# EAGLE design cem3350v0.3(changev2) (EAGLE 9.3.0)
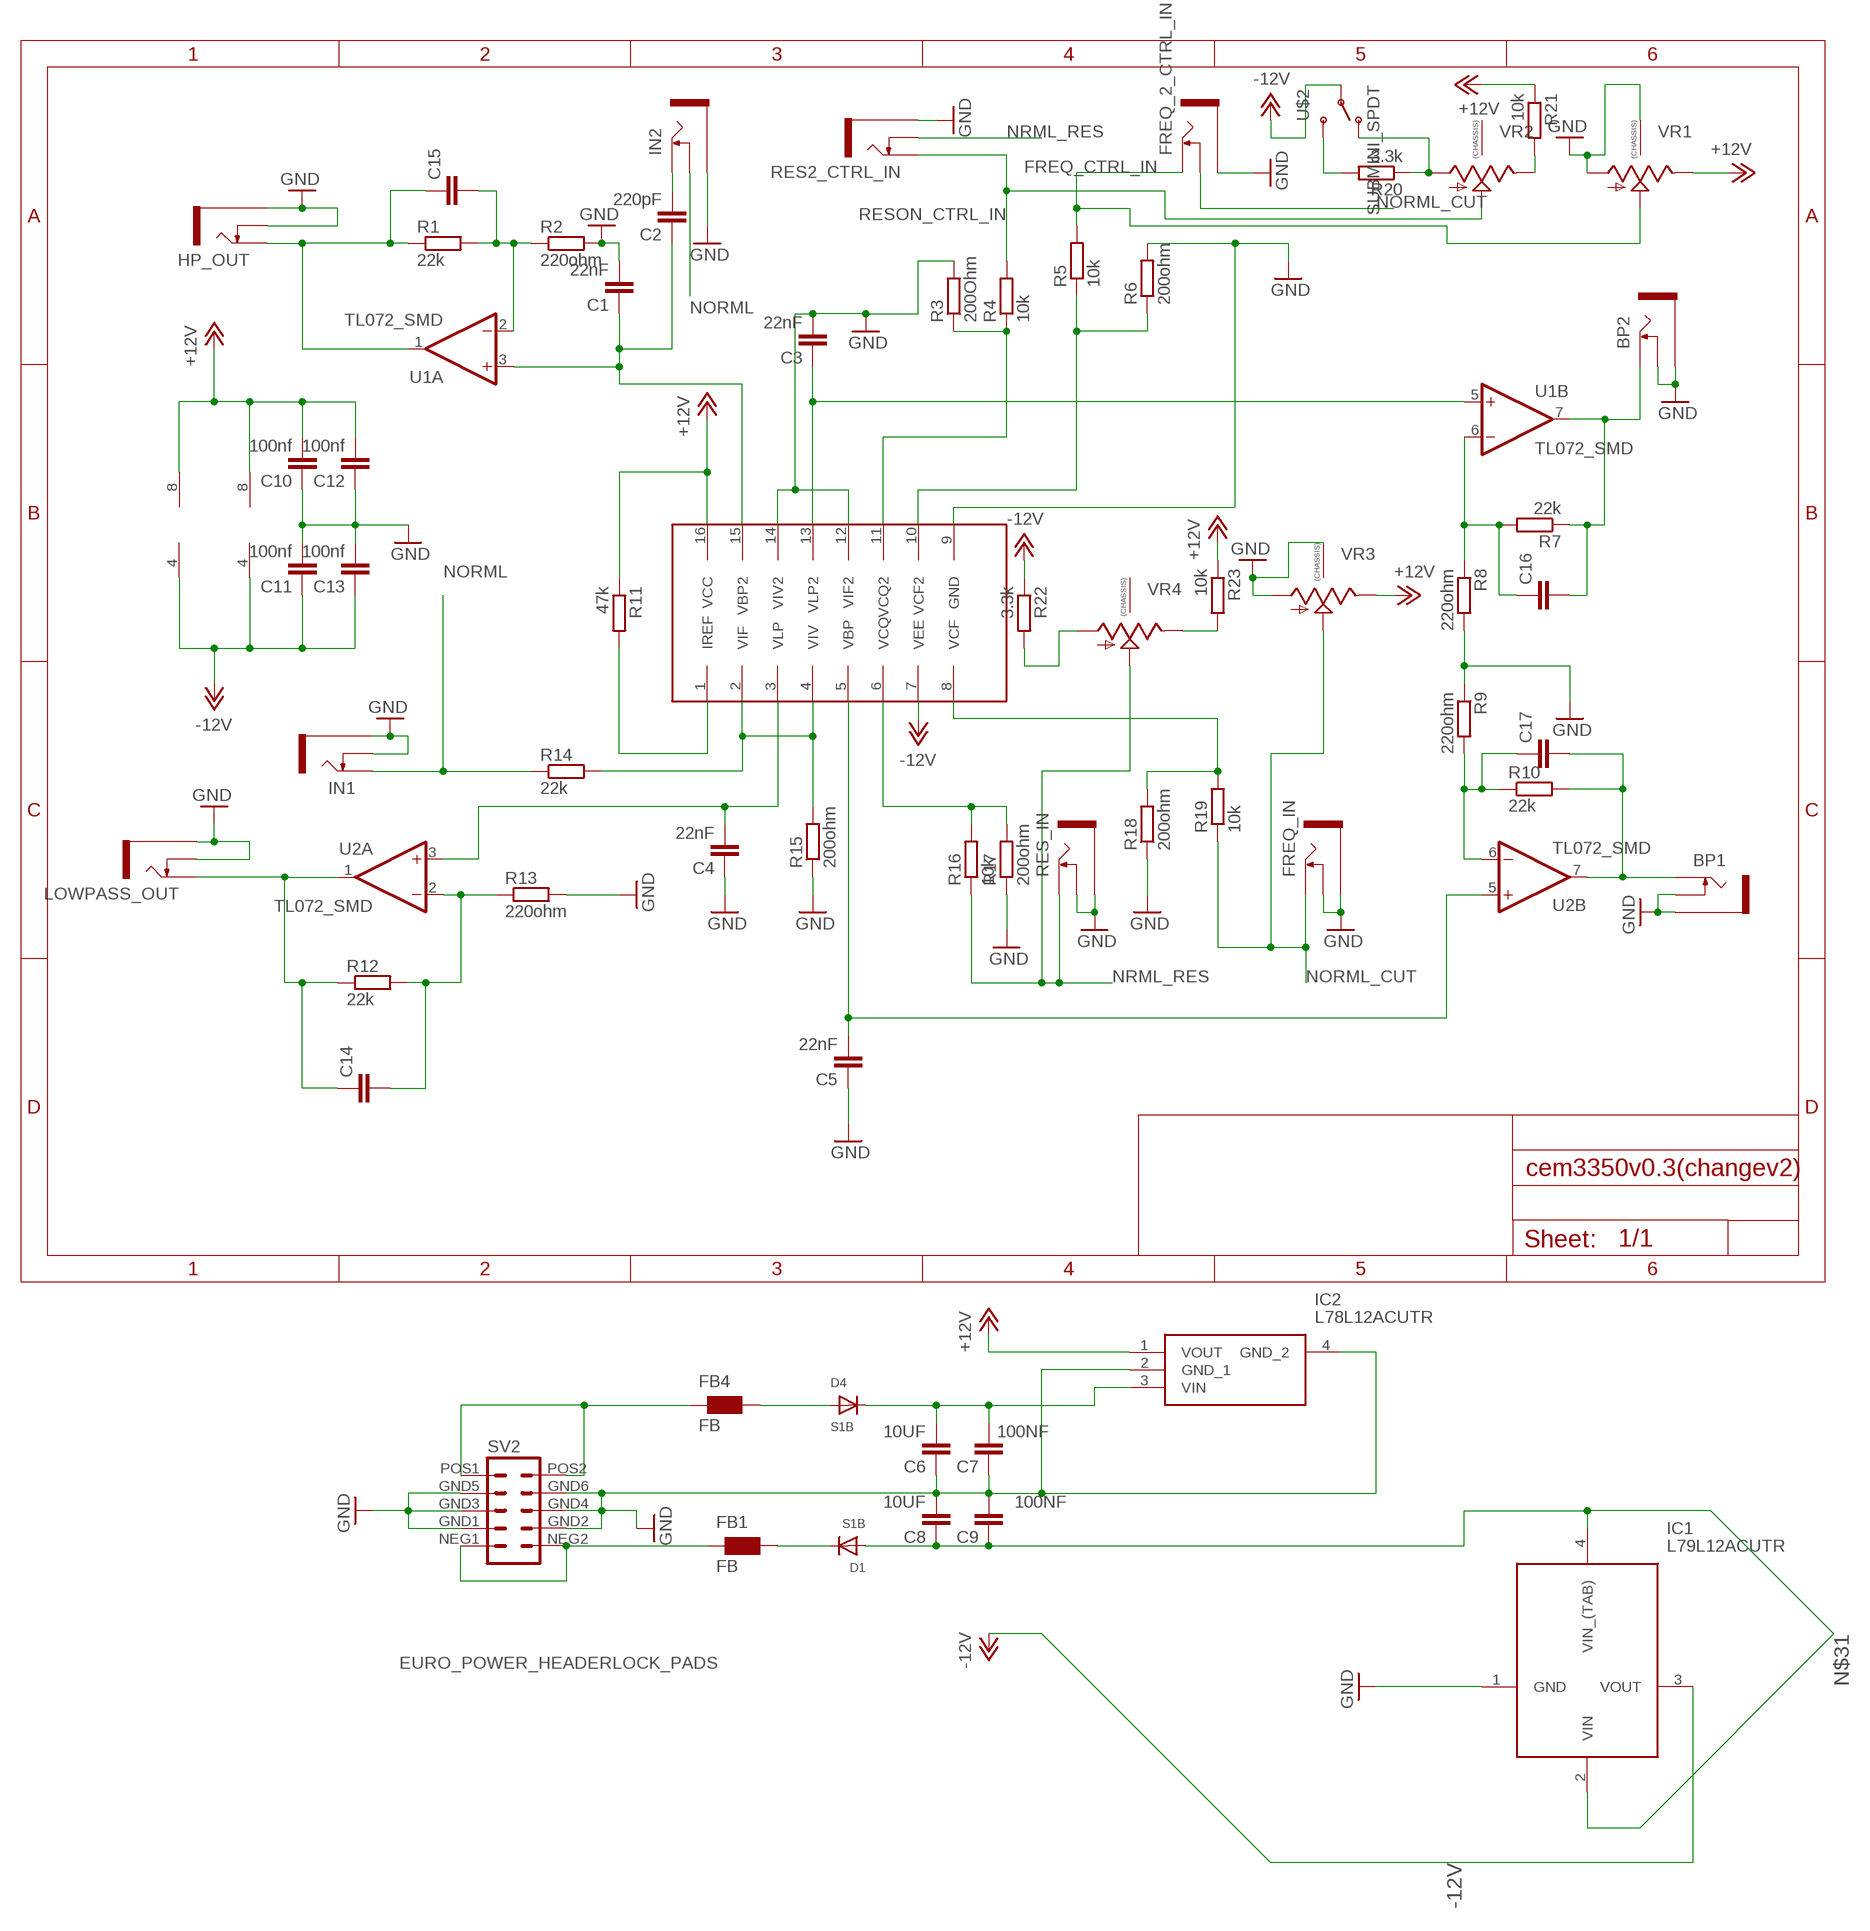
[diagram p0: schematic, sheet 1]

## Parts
BP1  THONKICONNNEW  [WQP-PJ301M-12_JACK]
BP2  THONKICONNNEW  [WQP-PJ301M-12_JACK]
C1  22nF  C-EUC0805  [C0805]
C2  220pF  C-EUC0805  [C0805]
C3  22nF  C-EUC0805  [C0805]
C4  22nF  C-EUC0805  [C0805]
C5  22nF  C-EUC0805  [C0805]
C6  10UF  C-EUC0805  [C0805]
C7  100NF  C-EUC0603  [C0603]
C8  10UF  C-EUC0805  [C0805]
C9  100NF  C-EUC0603  [C0603]
C10  100nf  C-EUC0603  [C0603]
C11  100nf  C-EUC0603  [C0603]
C12  100nf  C-EUC0603  [C0603]
C13  100nf  C-EUC0603  [C0603]
C14  C-EU050-024X044  [C050-024X044]
C15  C-EU050-024X044  [C050-024X044]
C16  C-EU050-024X044  [C050-024X044]
C17  C-EU050-024X044  [C050-024X044]
D1  S1B  [SMADIODE]
D4  S1B  [SMADIODE]
FB1  FB  FERRITE_BEAD_0603  [WUERTH-ELEKTRONIK_0603]
FB4  FB  FERRITE_BEAD_0603  [WUERTH-ELEKTRONIK_0603]
FREQ_2_CTRL_IN  THONKICONNNEW  [WQP-PJ301M-12_JACK]
FREQ_IN  THONKICONNNEW  [WQP-PJ301M-12_JACK]
HP_OUT  THONKICONNNEW  [WQP-PJ301M-12_JACK]
IC1  L79L12ACUTR  [ST-SOT-89]
IC2  L78L12ACUTR  [L78L12ACUTR]
IN1  THONKICONNNEW  [WQP-PJ301M-12_JACK]
IN2  THONKICONNNEW  [WQP-PJ301M-12_JACK]
LOWPASS_OUT  THONKICONNNEW  [WQP-PJ301M-12_JACK]
R1  22k  R-EU_R0805  [R0805]
R2  220ohm  R-EU_R0805  [R0805]
R3  200Ohm  R-EU_R0805  [R0805]
R4  10k  R-EU_R0805  [R0805]
R5  10k  R-EU_R0805  [R0805]
R6  200ohm  R-EU_R0805  [R0805]
R7  22k  R-EU_R0805  [R0805]
R8  220ohm  R-EU_R0805  [R0805]
R9  220ohm  R-EU_R0805  [R0805]
R10  22k  R-EU_R0805  [R0805]
R11  47k  R-EU_R0805  [R0805]
R12  22k  R-EU_R0805  [R0805]
R13  220ohm  R-EU_R0805  [R0805]
R14  22k  R-EU_R0805  [R0805]
R15  200ohm  R-EU_R0805  [R0805]
R16  10k  R-EU_R0805  [R0805]
R17  200ohm  R-EU_R0805  [R0805]
R18  200ohm  R-EU_R0805  [R0805]
R19  10k  R-EU_R0805  [R0805]
R20  3.3k  RESISTOR7MM  [7MM_RESISTOR]
R21  10k  RESISTOR7MM  [7MM_RESISTOR]
R22  3.3k  RESISTOR7MM  [7MM_RESISTOR]
R23  10k  RESISTOR7MM  [7MM_RESISTOR]
RES2_CTRL_IN  THONKICONNNEW  [WQP-PJ301M-12_JACK]
RES_IN  THONKICONNNEW  [WQP-PJ301M-12_JACK]
SV2  EURO_POWER_HEADERLOCK_PADS  [EURO_PWR_HEADER_LOCK]
U1  TL072_SMD  [SO08]
U2  TL072_SMD  [SO08]
U$1  CEM3350  [DIL16]
U$2  SUBMINI_SPDT  [SUBMINI_TOGGLE]
VR1  9MM_SNAP-IN_POT_CHASSIS  [9MM_SNAP-IN_POT]
VR2  9MM_SNAP-IN_POT_CHASSIS  [9MM_SNAP-IN_POT]
VR3  9MM_SNAP-IN_POT_CHASSIS  [9MM_SNAP-IN_POT]
VR4  9MM_SNAP-IN_POT_CHASSIS  [9MM_SNAP-IN_POT]

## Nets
+12V: C10.2 C12.2 IC2.1(VOUT) R11.1 R21.1 R23.1 U1.8(P:V+) U2.8(P:V+) U$1.16(VCC) VR1.3(E) VR3.3(E)
-12V: C11.1 C13.1 IC1.3(VOUT) R22.1 U1.4(P:V-) U2.4(P:V-) U$1.7(VEE) U$2.COM(COMMON)
FREQ_CTRL_IN: FREQ_2_CTRL_IN.P$1_TIP(TIP) R5.2 VR1.2(S)
GND: BP1.P$2_SWITCH(SWITCH) BP1.P$3_SLEEVE(SLEEVE) BP2.P$2_SWITCH(SWITCH) BP2.P$3_SLEEVE(SLEEVE) C1.2 C3.2 C4.1 C5.1 C6.1 C7.1 C8.2 C9.2 C10.1 C11.2 C12.1 C13.2 FREQ_2_CTRL_IN.P$3_SLEEVE(SLEEVE) FREQ_IN.P$2_SWITCH(SWITCH) FREQ_IN.P$3_SLEEVE(SLEEVE) HP_OUT.P$2_SWITCH(SWITCH) HP_OUT.P$3_SLEEVE(SLEEVE) IC1.1(GND) IC2.2(GND_1) IC2.4(GND_2) IN1.P$2_SWITCH(SWITCH) IN1.P$3_SLEEVE(SLEEVE) IN2.P$3_SLEEVE(SLEEVE) LOWPASS_OUT.P$2_SWITCH(SWITCH) LOWPASS_OUT.P$3_SLEEVE(SLEEVE) R2.2 R3.2 R6.2 R8.2 R9.1 R13.2 R15.1 R17.1 R18.1 RES2_CTRL_IN.P$3_SLEEVE(SLEEVE) RES_IN.P$2_SWITCH(SWITCH) RES_IN.P$3_SLEEVE(SLEEVE) SV2.GND1 SV2.GND2 SV2.GND3 SV2.GND4 SV2.GND5 SV2.GND6 U$1.9(GND) U$1.12(VIF2) U$1.14(VIV2) VR1.1(A) VR1.CHASSIS1 VR1.CHASSIS2 VR3.1(A) VR3.CHASSIS1 VR3.CHASSIS2
N$1: R11.2 U$1.1(IREF)
N$2: C15.2 R1.2 R2.1 U1.2(A:-IN)
N$3: C2.2 IN2.P$1_TIP(TIP)
N$4: R3.1 R4.1 U$1.11(VCQ2)
N$5: C1.1 C2.1 U1.3(A:+IN) U$1.15(VBP2)
N$6: C16.1 R7.2 R8.1 U1.6(B:-IN)
N$7: C3.1 U1.5(B:+IN) U$1.13(VLP2)
N$8: C15.1 HP_OUT.P$1_TIP(TIP) R1.1 U1.1(A:OUT)
N$9: BP2.P$1_TIP(TIP) C16.2 R7.1 U1.7(B:OUT)
N$10: R5.1 R6.1 U$1.10(VCF2)
N$11: FB1.1 SV2.NEG1 SV2.NEG2
N$12: C17.1 R9.2 R10.1 U2.6(B:-IN)
N$13: BP1.P$1_TIP(TIP) C17.2 R10.2 U2.7(B:OUT)
N$14: R18.2 R19.2 U$1.8(VCF)
N$15: R16.2 R17.2 U$1.6(VCQ)
N$16: C5.2 U2.5(B:+IN) U$1.5(VBP)
N$17: R14.2 R15.2 U$1.2(VIF) U$1.4(VIV)
N$18: FB4.1 SV2.POS1 SV2.POS2
N$19: C4.2 U2.3(A:+IN) U$1.3(VLP)
N$20: C14.2 R12.2 R13.1 U2.2(A:-IN)
N$21: C14.1 LOWPASS_OUT.P$1_TIP(TIP) R12.1 U2.1(A:OUT)
N$22: D4.A FB4.2
N$23: D1.C FB1.2
N$24: R21.2 VR2.3(E)
N$25: R20.1 U$2.1(O) VR2.1(A)
N$26: R20.2 U$2.3(S)
N$27: R22.2 VR4.1(A)
N$28: R23.2 VR4.3(E)
N$29: C6.2 C7.2 D4.C IC2.3(VIN)
N$31: C8.1 C9.1 D1.A IC1.2(VIN) IC1.4(VIN_(TAB))
NORML: IN1.P$1_TIP(TIP) IN2.P$2_SWITCH(SWITCH) R14.1
NORML_CUT: FREQ_2_CTRL_IN.P$2_SWITCH(SWITCH) FREQ_IN.P$1_TIP(TIP) R19.1 VR3.2(S)
NRML_RES: R16.1 RES2_CTRL_IN.P$2_SWITCH(SWITCH) RES_IN.P$1_TIP(TIP) VR4.2(S)
RESON_CTRL_IN: R4.2 RES2_CTRL_IN.P$1_TIP(TIP) VR2.2(S)
Unconnected: VR2.CHASSIS1 VR2.CHASSIS2 VR4.CHASSIS1 VR4.CHASSIS2

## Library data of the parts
BP1 BP2 FREQ_2_CTRL_IN FREQ_IN HP_OUT IN1 IN2 LOWPASS_OUT RES2_CTRL_IN RES_IN = MusicThingModular:THONKICONN: 3.5mm socket for Eurorack modular synths
C1-C17 = rcl:C-EU: CAPACITOR, European symbol; SPICEPREFIX: C
D1 D4 = Electrosmith-Semiconductors:S1B; BIN#: 12-006; IPN: S1B; MPN: S1B; PACKAGE: SMA
FB1 FB4 = Electrosmith-Passives:FERRITE_BEAD: SMD EMI Suppression Ferrite Beads; BIN#: 8-047; IPN: FB R0603; MPN: MI0603J601R-10; PACKAGE: R0603
IC1 = MusicThingModular:L79L12ACUTR: L79L12ACUTR, Voltage Regulator, Negative 0.1A -12 V, +/-5%, 4-Pin SOT-89 Source: Datasheet; ARROW_PART_NUMBER: L79L12ACUTR; ARROW_PRICE-STOCK: https://www.arrow.com/en/products/l79l12acutr/stmicroelectronics; DESCRIPTION: L79L12ACUTR, Voltage Regulator, Negative 0.1A -12 V, +/-5%, 4-Pin SOT-89; HEIGHT: mm; MANUFACTURER_NAME: STMicroelectronics; MANUFACTURER_PART_NUMBER: L79L12ACUTR; MOUSER_PART_NUMBER: 511-L79L12ACU-TR; MOUSER_PRICE-STOCK: https://www.mouser.co.uk/ProductDetail/STMicroelectronics/L79L12ACUTR?qs=t0%252BWbrArM4MWNjS3Dlb5lQ%3D%3D
IC2 = MusicThingModular:L78L12ACUTR: Linear Voltage Regulators 12V 0.1A Positive Source: Datasheet; ARROW_PART_NUMBER: L78L12ACUTR; ARROW_PRICE-STOCK: https://www.arrow.com/en/products/l78l12acutr/stmicroelectronics; DESCRIPTION: Linear Voltage Regulators 12V 0.1A Positive; HEIGHT: 1.6mm; MANUFACTURER_NAME: STMicroelectronics; MANUFACTURER_PART_NUMBER: L78L12ACUTR; MOUSER_PART_NUMBER: 511-L78L12ACU; MOUSER_PRICE-STOCK: https://www.mouser.co.uk/ProductDetail/STMicroelectronics/L78L12ACUTR?qs=lsQ%2Fasl43rq%252BGNm5TGwtyg%3D%3D
R1-R19 = rcl:R-EU_: RESISTOR, European symbol; SPICEPREFIX: R
R20-R23 = MusicThingModular:RESISTOR: Standard resistor, various versions
SV2 = MusicThingModular:EURO_POWER_HEADER: Power Header 10 pin power header for Eurorack Power Supplies Variants with fatter pads for easier soldering, and the LOCK variant which has 5mil offset pins to hold the component in place before soldering
U1 U2 = MusicThingModular:TL072: Generic Dual Op Amp
U$1 = CEM:CEM3350
U$2 = MusicThingModular:SUBMINI_SPDT
VR1-VR4 = MusicThingModular:9MM_SNAP-IN_POT_CHASSIS: 9mm vertical snap-in pot, Alpha / Panasonic style, with a connection to the metal chassis for grounding

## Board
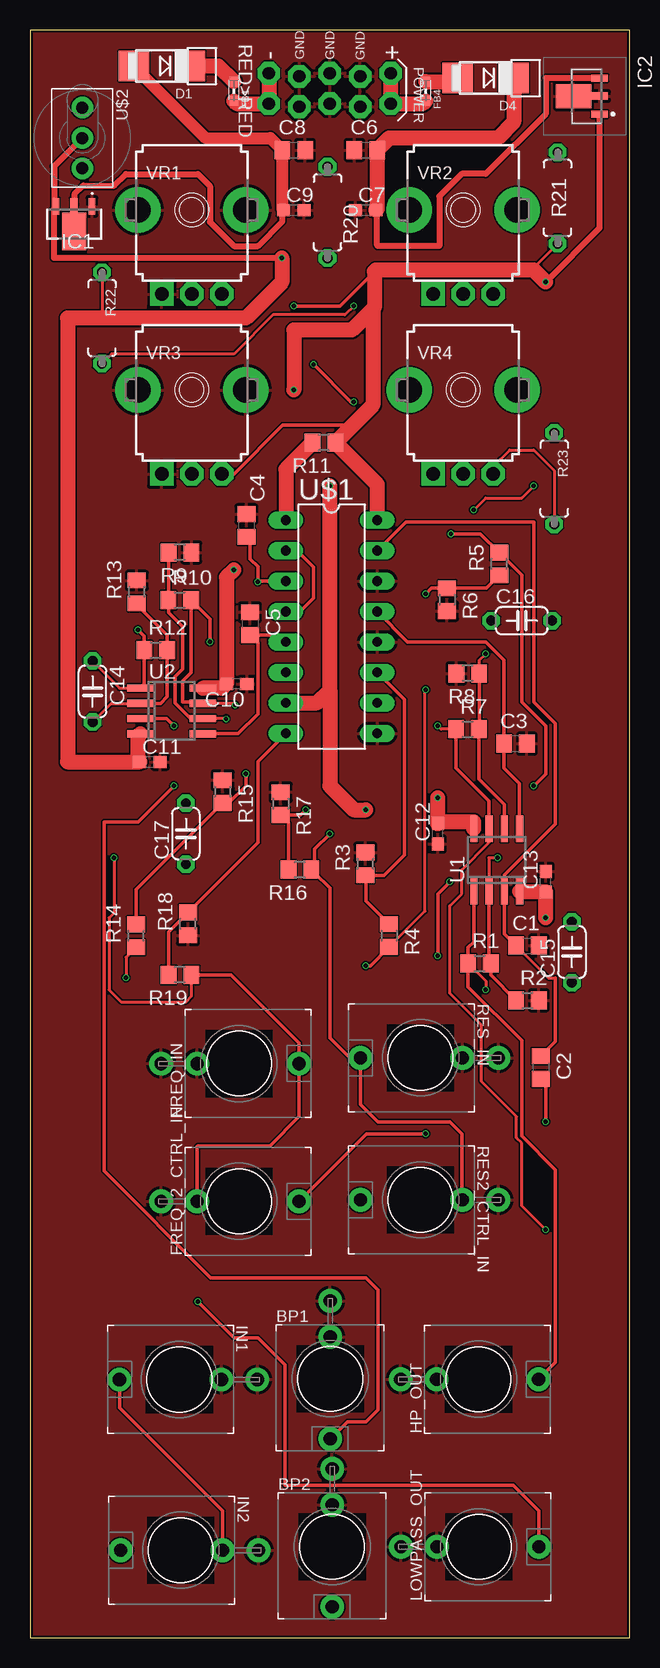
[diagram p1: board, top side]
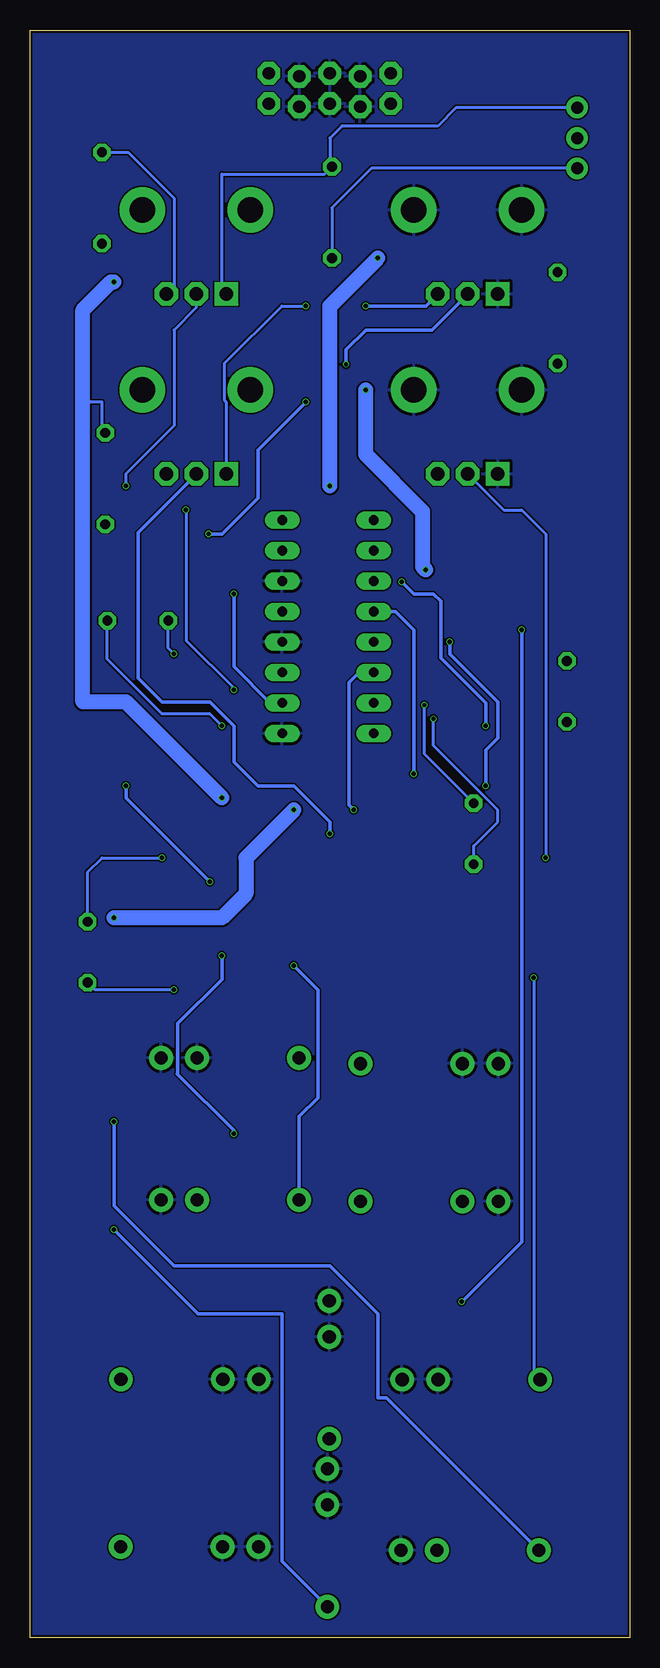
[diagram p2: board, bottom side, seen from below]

Size 50 x 134 mm. Coordinates in mm from the lower left corner, seen from the top.
Outline: 0,0 50,0 50,134 0,134 0,0
Copper layers (1*16): Top 0.035mm / dielectric 1.6mm / Bottom 0.035mm
Design rules "jlcpcb-2layers": minimum track width 5mil, minimum drill 0.3mm, track to track 5mil, track to pad 5mil, pad to pad 5mil, via to via 5mil, smd to smd 5mil, copper to edge 0.2mm, drill to drill 6mil, minimum pad ring 10mil, minimum via ring 3mil, stop-mask expansion 4mil, vias tented up to drill 0mil, thermal gap 10mil

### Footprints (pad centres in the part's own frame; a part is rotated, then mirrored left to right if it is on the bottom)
WQP-PJ301M-12_JACK = drill 1.1: P$1_TIP 0,5; P$2_SWITCH 0,-3.5; P$3_SLEEVE 0,-6.5
C0805 = smd 1.3 x 1.5: 1 -0.95,0; 2 0.95,0
C0603 = smd 1.1 x 1: 1 -0.85,0; 2 0.85,0
C050-024X044 = drill 0.813 octagon: 1 -2.54,0; 2 2.54,0
SMADIODE = smd 2.54 x 2.54: A 2.349,0; C -2.349,0
WUERTH-ELEKTRONIK_0603 = smd 0.85 x 0.7: 1 -0.9,0; 2 0.7,0
ST-SOT-89 = smd 0.57 x 1.4: 1 -1.5,-1.475; 3 1.5,-1.475 | smd 0.65 x 1.2: 2 0,-1.575 | smd 2 x 3.15: 4 0,0.6
L78L12ACUTR = smd 0.57 x 1.4: 1 -1.5,0; 3 1.5,0 | smd 0.65 x 1.4: 2 0,0 | smd 2 x 2.95: 4 0,2.175
R0805 = smd 1.3 x 1.5: 1 -0.95,0; 2 0.95,0
7MM_RESISTOR = drill 0.813 octagon: 1 -3.81,0; 2 3.81,0
EURO_PWR_HEADER_LOCK = drill 1.016 pad 1.88 octagon: GND1 -2.54,1.143; GND2 -2.54,-1.397; GND3 0,1.397; GND4 0,-1.143; GND5 2.54,1.143; GND6 2.54,-1.397; NEG1 -5.08,1.397; NEG2 -5.08,-1.143; POS1 5.08,1.397; POS2 5.08,-1.143
SO08 = smd 0.6 x 2.2: 1 -1.905,-2.6; 2 -0.635,-2.6; 3 0.635,-2.6; 4 1.905,-2.6; 5 1.905,2.6; 6 0.635,2.6; 7 -0.635,2.6; 8 -1.905,2.6
DIL16 = drill 0.813 long: 1 -8.89,-3.81; 2 -6.35,-3.81; 3 -3.81,-3.81; 4 -1.27,-3.81; 5 1.27,-3.81; 6 3.81,-3.81; 7 6.35,-3.81; 8 8.89,-3.81; 9 8.89,3.81; 10 6.35,3.81; 11 3.81,3.81; 12 1.27,3.81; 13 -1.27,3.81; 14 -3.81,3.81; 15 -6.35,3.81; 16 -8.89,3.81
SUBMINI_TOGGLE = drill 1 pad 1.422: 1 -2.54,0; 3 2.54,0; COM 0,0
9MM_SNAP-IN_POT = drill 1.1 square: 1 -2.5,-7 | drill 1.1 octagon: 2 0,-7; 3 2.5,-7 | drill 2.1 pad 2.794: CHASSIS1 -4.5,0; CHASSIS2 4.5,0

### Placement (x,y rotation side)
BP1  25.04,21.57 180 top
BP2  25.2,7.57 180 top
C1  41.49,57.67 0 top
C2  42.59,47.51 270 top
C3  40.49,74.51 0 top
C4  18.04,92.7 270 top
C5  18.35,84.51 270 top
C6  28,124 0 top
C7  28,119 0 top
C8  22,124 0 top
C9  22,119 0 top
C10  17.24,79.49 180 top
C11  10,73 0 top
C12  34,67 90 top
C13  43,63 90 top
C14  5.22,78.86 270 top
C15  45.19,57.13 90 top
C16  41.01,84.77 0 top
C17  13,67 90 top
D1  11,131 180 top
D4  38,130 180 top
FB1  17,129 90 top
FB4  33,129 90 top
FREQ_2_CTRL_IN  17.43,36.36 270 top
FREQ_IN  17.43,47.84 270 top
HP_OUT  37.41,21.53 270 top
IC1  3.67,117.81 180 top
IC2  47.51,128.49 90 top
IN1  12.46,21.5 90 top
IN2  12.57,7.28 90 top
LOWPASS_OUT  37.43,7.56 270 top
R1  37.49,56.19 0 top
R2  41.49,53.11 0 top
R3  27.97,64.49 90 top
R4  29.95,58.51 270 top
R5  39.13,89.49 90 top
R6  34.79,86.51 270 top
R7  36.49,75.71 0 top
R8  36.51,80.37 180 top
R9  12.51,90.45 180 top
R10  12.49,86.47 0 top
R11  24.51,99.61 180 top
R12  10.49,82.31 0 top
R13  8.91,87.16 90 top
R14  8.85,58.49 90 top
R15  16.07,70.51 270 top
R16  22.51,64.01 180 top
R17  20.91,69.51 270 top
R18  13.17,59.49 90 top
R19  12.51,55.25 180 top
R20  24.81,118.8 270 top
R21  44,120 90 top
R22  6,110 270 top
R23  43.73,96.61 270 top
RES2_CTRL_IN  32.57,36.48 90 top
RES_IN  32.57,48.32 90 top
SV2  25,129 0 top
U1  38.92,64.81 0 top
U2  11.81,77.24 270 top
U$1  25.15,84.26 270 top
U$2  4.37,125 270 top
VR1  13.49,119 0 top
VR2  36.12,119 0 top
VR3  13.49,104 0 top
VR4  36.12,104 0 top

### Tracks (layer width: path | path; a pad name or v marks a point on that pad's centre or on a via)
+12V  (via drill 0.35)
  Top 0.254: R21.1 42,114.19 42,114
  Top 0.305: 28.85,114 28.72,113.87 25.85,111 v22,111 | 26.93,101.08 21.07,101.08 17,97 VR3.3
  Top 0.508: v43,113 47.51,117.51 IC2.1
  Top 1.27: U1.8 37,67.42 37,68 34.15,68 C12.2 v34,70 | U2.8 16.04,79.14 C10.2 16.39,88.39 v17,89 | U$1.16 28.96,96.11 R11.1 26.93,101.08 28.6,102.75 28.6,110.75 | 28.72,113.87 28.72,110.87 28.6,110.75 | v43,113 42,114 28.85,114 | 28.6,110.75 26.85,109 22,109 v22,104
  Bottom 0.254: R23.1 44,100.69 44,103 45.6,103
  Bottom 0.305: v22,111 16.99,111 VR1.3
  Bottom 1.27: v34,70 42,78 45.6,78 45.6,103 45.6,110.65 43.25,113 v43,113 | v22,104 22.02,103.98 22.02,98.64 17.25,93.87 17.25,89.25 v17,89
-12V  (via drill 0.35)
  Top 0.254: R22.1 6,110
  Top 0.508: v21,115 2,115 2,119.12 | 2,119.12 IC1.3 | U$2.COM 2,122.64 2,119.12
  Top 1.27: U1.4 40.88,62.15 C13.1 v43,60 | U2.4 9,75.12 9,73.15 C11.1 3.14,73 3.14,110 6,110 18,110 21,113 v21,115 | U$1.7 23.91,77.91 25,79 | 25,79 v25,96 | 25,79 25,71 27,69 v28,69
  Bottom 1.27: v25,96 25,111 v21,115 | v28,69 32,65 32,62 34,60 v43,60
FREQ_CTRL_IN  (via drill 0.35)
  Top 0.305: v23.64,106.13 26.76,103 v27,103 | v35.09,92 37.57,92 R5.2 41,88.57 41,78 43,76 43,72 v42,71 | FREQ_2_CTRL_IN.P$1_TIP 28.07,42 v33,42 | v34,56.83 34,62 v35,63
  Bottom 0.305: VR1.2 16.49,109 22,109 23.64,107.36 v23.64,106.13 | v27,103 31,99 31,95 34,92 v35.09,92 | v42,71 42,70 v35,63 | v33,42 33,42.25 37.75,47 37.69,47 37.69,51.17 34,54.86 v34,56.83
GND
  pour Top: 0,134 51,134 51,0 0,0
  pour Bottom: 0,135 50,135 50,0 0,0
N$1
  Top 1.27: R11.2 21.34,97.39 U$1.1
N$2  (via drill 0.35)
  Top 0.254: v39,65 38.25,65 38.25,62.24 U1.2
  Top 0.305: R2.1 38.44,55.21 R1.2 38.28,56.34 U1.2
  Bottom 0.254: C15.2 45.19,63.81 44,65 v39,65
N$3  (via drill 0.35)
  Top 0.305: v43,43 43,46.15 C2.2
  Bottom 0.305: IN2.P$1_TIP 20.29,20 21,20 21,27 25,31 38,31 43,36 v43,43
N$4
  Top 0.305: U$1.11 31.24,78.17 31.24,65.24 29.54,63.54 28,63.54 | 28,63.54 R3.1 | R4.1 28,61.41 28,63.54
N$5
  Top 0.254: C1.1 43.21,55 43.83,55
  Top 0.305: C1.1 39.55,58.66 U1.3 39.55,63.55 43.83,67.83 43.83,76.17 42,78 42,93 31.35,93 U$1.15 | C2.1 43.83,49.7 43.83,55
N$6  (via drill 0.35)
  Top 0.254: R8.1 37.46,81.46 v38,82
  Top 0.305: R8.1 37.46,75.73 R7.2 37.44,71.56 39.55,69.44 U1.6
  Bottom 0.254: v38,82 38.47,82.47 C16.1
N$7
  Top 0.305: U1.5 40.83,71.17 39.54,72.46 C3.1 39.54,81.46 38,83 31.49,83 U$1.13
N$8  (via drill 0.35)
  Top 0.254: R1.1 38,54.73 v38,54
  Top 0.305: U1.1 37,62.2 37,58 36.54,57.54 R1.1 36.54,54.22 41,49.76 41,41.83 43.83,39 43.83,22.95 HP_OUT.P$1_TIP
  Bottom 0.254: v38,54 44.6,54 C15.1
N$9  (via drill 0.35)
  Top 0.254: v43,34 41,36 41,41.22 40.57,41.65 40.57,43.43 37.64,46.36 37.64,51.05 35,53.69 35,61 36,62 36,64 38.28,66.28 38.28,68 | R7.1 34.29,75.71 v34,76
  Top 0.305: U1.7 38.28,68 38.28,69.72 35.54,72.46 R7.1
  Bottom 0.254: v34,76 35,77 39,77 43.55,81.55 C16.2
  Bottom 0.305: BP2.P$1_TIP 29,6.37 29,27 36,27 v43,34
N$10  (via drill 0.35)
  Top 0.305: R5.1 38.05,87.46 R6.1 33.46,87.46 v33,87
  Bottom 0.305: U$1.10 29.96,77.91 33,80.95 v33,87
N$11
  Top 1.27: SV2.NEG1 SV2.NEG2 17.24,127.86 FB1.1
N$12  (via drill 0.35)
  Top 0.254: v16.35,76.58 16.33,76.61 14,76.61
  Top 0.305: R9.2 11.56,86.49 | 11.56,86.49 R10.1 | U2.6 14,76.61 13.39,76.61 12.11,77.89 12.11,80.11 12.75,80.75 12.75,84.25 11.56,85.44 11.56,86.49
  Bottom 0.254: C17.1 13,66 11,68 11,69 16.35,74.35 v16.35,76.58
N$13  (via drill 0.35)
  Top 0.254: v17.11,77.72 16.96,77.88 U2.7
  Top 0.305: U2.7 14.29,78 12.75,78 12.75,79.75 13.44,80.44 R10.2 15,84.91 v15,83 | BP1.P$1_TIP 26.47,18 28,18 29,19 29,29 28,30 15.06,30 6.17,38.89 6.17,68 9,68 v12,71
  Bottom 0.254: C17.2 17.11,73.65 v17.11,77.72
  Bottom 0.305: v15,83 15,82 11,78 11,75 12,74 v12,71
N$14
  Top 0.305: U$1.8 19,73.03 19,66.27 R18.2 11.56,58.83 R19.2
N$15  (via drill 0.35)
  Top 0.305: v23,69 22.56,68.56 R17.2 21.56,67.91 R16.2
  Bottom 0.305: U$1.6 22.55,80.45 23.38,79.62 23.38,69.38 v23,69
N$16
  Top 0.305: U$1.5 20.77,83.56 C5.2 19,82.91 19,77 17.34,75.33 U2.5
N$17  (via drill 0.35)
  Top 0.305: U$1.4 22.53,85.53 23.64,86.64 23.64,89.24 22.26,90.61 U$1.2 | v18,72 18,71 16.56,69.56 R15.2 8.85,62.34 R14.2
  Bottom 0.305: U$1.4 19.53,85.53 18,84 v18,72
N$18
  Top 1.27: SV2.POS1 SV2.POS2 32.76,127.86 FB4.1
N$19  (via drill 0.35)
  Top 0.305: U2.3 11.39,76.61 v12,76 | C4.2 18.36,91.42 18.36,89.91 19,89.27 v19,88 19.07,88.07 U$1.3
  Bottom 0.305: v12,76 12,77.91 15.75,81.65 15.75,86.38 16.36,87 18,87 v19,88
N$20
  Top 0.254: C14.2 6.78,77.88 U2.2
  Top 0.305: U2.2 10.88,77.88 11.44,78.44 R12.2 11.44,83.56 8.91,86.09 R13.1
N$21  (via drill 0.35)
  Top 0.254: C14.1 7.48,79.14 U2.1
  Top 0.305: U2.1 9.54,79.47 R12.1 9.54,83.46 v9,84 | v14,28 17,25 19,25 21.25,22.75 21.25,12.71 40.29,12.71 42.43,10.57 LOWPASS_OUT.P$1_TIP
  Bottom 0.305: v9,84 9,33 v14,28
N$22
  Top 1.27: FB4.2 35.35,129.7 D4.A
N$23
  Top 1.27: FB1.2 15.7,131 D1.C
N$24
  Bottom 0.254: R21.2 41.81,123.81 38,120 38,112.62 VR2.3
N$25
  Bottom 0.254: U$2.1 14.46,127.54 16,126 24,126 25,125 25,122.79 R20.1 25.42,122 34,122 34,112.38 VR2.1
N$26
  Bottom 0.254: U$2.3 21.54,122.46 24.81,119.19 R20.2
N$27  (via drill 0.35)
  Top 0.254: v27,111 26.25,110.25 20.25,110.25 17,107 6.81,107 R22.2
  Bottom 0.254: VR4.1 33.62,102.97 33.76,103.11 33.76,106.24 29,111 v27,111
N$28
  Top 0.254: VR4.3 38.62,97.62 40,99 42,99 43.73,97.28 R23.2
N$29
  Top 0.508: IC2.3 43,130 43,127 38.02,122.02 36.02,122.02 34.13,120.13 34.13,116 29,116 28.95,116.05 28.95,120
  Top 1.27: D4.C 40.35,126.35 39,125 29.95,125 C6.2 28.95,120 28.95,119.1 C7.2
N$31
  Top 0.508: 21.05,119.1 21.05,118.05 19,116 17,116 15,118 15,121 14,122 8,122 7.03,121.03 4.45,121.03 3.71,120.29 3.71,119.5 3.75,119.46 IC1.2 IC1.4
  Top 1.016: D1.A 14.65,125 20.05,125 C8.1 21.05,119.1 C9.1
NORML  (via drill 0.35)
  Top 0.254: v8,55 8,56.69 R14.1
  Top 0.305: IN2.P$2_SWITCH 16.07,10.55 7.46,19.16 IN1.P$1_TIP
  Bottom 0.254: IN1.P$1_TIP 7.97,22.01 7.97,54.97 v8,55
NORML_CUT  (via drill 0.35)
  Top 0.254: v7,65 7,60.38 6.6,59.98 6.6,54 7.6,53 13,53 13.46,53.46 R19.1
  Top 0.305: R19.1 16.75,55.25 22.43,49.57 FREQ_IN.P$1_TIP 22.43,43.43 20,41 14,41 13.93,40.93 FREQ_2_CTRL_IN.P$2_SWITCH
  Bottom 0.254: VR3.2 10.49,94 9,94 7,92 v7,65
NRML_RES  (via drill 0.35)
  Top 0.305: R16.1 23.73,63.73 | 23.73,63.73 25,62.47 25,50 26.68,48.32 RES_IN.P$1_TIP 27.57,44.43 29,43 35,43 36,42 36,36.55 RES2_CTRL_IN.P$2_SWITCH | 23.73,63.73 23.73,65.73 v25,67
  Bottom 0.305: VR4.2 41,92.12 41,80 39,78 35,78 33,76 33,73 31,71 28,71 25,68 v25,67
RESON_CTRL_IN  (via drill 0.35)
  Top 0.254: R4.2 32.94,60.55 32.94,78.94 v33,79 | v37,94 38,95 41,95 v42,96
  Top 0.305: R4.2 28.39,56 v28,56
  Bottom 0.254: v33,79 33,79.13 36.97,83.09 36.97,93.97 v37,94 | v42,96 42,97.02 38,101.02 38,109 36.12,110.88 VR2.2
  Bottom 0.305: RES2_CTRL_IN.P$1_TIP 27.57,43.43 26,45 26,54 v28,56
